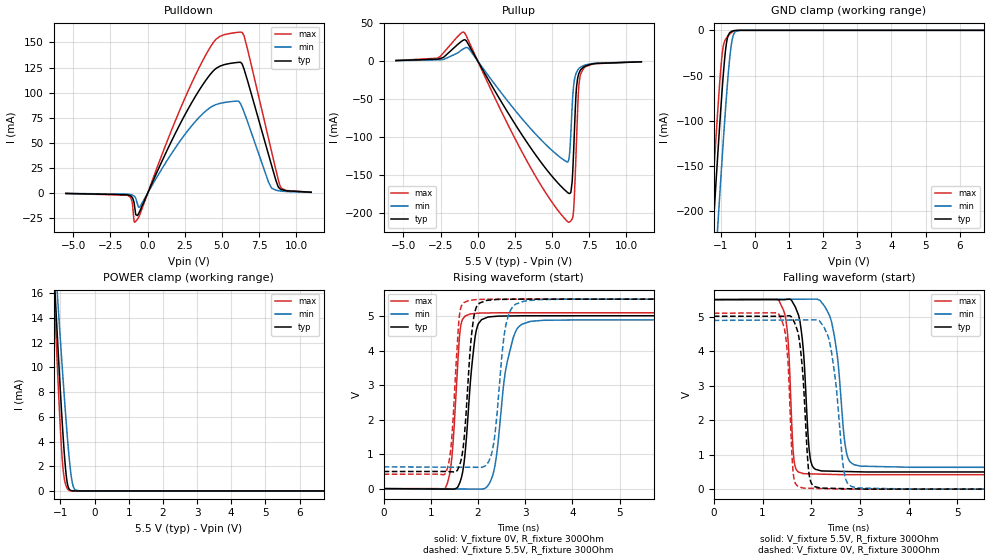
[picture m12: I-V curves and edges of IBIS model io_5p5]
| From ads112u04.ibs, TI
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|   io_5p5 Model
[Model]   io_5p5
Model_type   I/O
Polarity   Non-Inverting
Enable   Active-Low
Vinl = 1.65
Vinh = 3.85
Vmeas = 2.75
Vref = 0
Cref = 2pF
Rref = 100000
|   typ   min   max
C_comp   1.31716E-12   1.299E-12   1.3233E-12
|C_comp_pullup   9.8999E-13   9.67468E-13   1.02241E-12
|C_comp_pulldown   9.99226E-13   9.80937E-13   1.00378E-12
[Model spec]
|subparameter
Vinl   1.65   1.6497   1.6503
Vinh   3.85   3.8493   3.8507
| Where Nom  PVT is Nominal Process, 5.5V, 27C
|   Fast PVT is Strong Process,  5.501V, -40C
|   Slow PVT is Weak Process,   5.499, 125C
[Voltage Range]   5.5   5.499   5.501
[Temperature Range]   27   125   -40
[Pullup Reference]   5.5   5.499   5.501
[Pulldown Reference]   -0   -0   -0
[Power Clamp Reference]   5.5   5.499   5.501
[GND Clamp Reference]   0   0   0
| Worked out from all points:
|   slope of the pulldown table from 0 to 0.825 V, typ, clamps not added: 30.1 ohm
|   slope of the pullup table from 0 to 0.825 V, typ, clamps not added: 29 ohm
|   GND clamp passes 1 mA (typ) near -0.67 V on its own axis
|   POWER clamp passes 1 mA (typ) near -0.82 V on its own axis
|   falling waveform, V_fixture 5.5V, R_fixture 300Ohm: 20-80 % time 134ps typ, 206ps min, 99.9ps max; typ from 5.5 V to 0.497 V
|   rising waveform, V_fixture 0V, R_fixture 300Ohm: 20-80 % time 180ps typ, 269ps min, 138ps max; typ from 0 V to 5.02 V
|   rising waveform, V_fixture 5.5V, R_fixture 300Ohm: 20-80 % time 158ps typ, 202ps min, 133ps max; typ from 0.497 V to 5.5 V
|   falling waveform, V_fixture 0V, R_fixture 300Ohm: 20-80 % time 137ps typ, 209ps min, 102ps max; typ from 5.02 V to 0 V
[Pulldown]
|   Voltage   I(typ)   I(min)   I(max)
-5.5V     -139.3uA   -99uA      -151.9uA
-1.375V   -1.389mA   -810uA     -1.838mA
-995.5mV  -5.059mA   -1.917mA   -13.97mA
-797.5mV  -21.25mA   -4.806mA   -27.92mA
-517mV    -17.41mA   -13.24mA   -20.88mA
3.938V    112.8mA    82.15mA    138.3mA
4.862V    126.3mA    89.35mA    155.9mA
6.248V    130.2mA    89.06mA    160.2mA
6.495V    122.9mA    80.2mA     155.9mA
8.129V    38.5mA     11.1mA     54.47mA
8.921V    4.291mA    2.335mA    6.881mA
11V       1.086mA    904uA      1.089mA
[GND Clamp]
|   Voltage   I(typ)   I(min)   I(max)
-5.5V     -3.028A    -3.1A      -2.983A
-1.359V   -306.6mA   -386.8mA   -256.2mA
-1.243V   -234.4mA   -314.6mA   -184mA
-1.21V    -214.1mA   -294.2mA   -163.7mA
-1.078V   -134.5mA   -213.7mA   -85.68mA
-946mV    -61.21mA   -136.3mA   -23.61mA
-880mV    -30.87mA   -99.68mA   -11.73mA
-814mV    -10.85mA   -65.7mA    -7.744mA
-731.5mV  -2.627mA   -29.97mA   -4.178mA
-649mV    -712.3uA   -8.24mA    -1.554mA
-385mV    -967.4nA   -10.5uA    -935.9nA
11V       0A         0A         0A
[Pullup]
|   Voltage   I(typ)   I(min)   I(max)
-5.5V     607.8uA    492.8uA    650.8uA
-2.712V   2.442mA    1.477mA    3.672mA
-913mV    27.96mA    16.59mA    37.83mA
3.311V    -107.4mA   -83.78mA   -132.1mA
6.133V    -174.7mA   -129mA     -212.7mA
6.347V    -159.6mA   -60.35mA   -208.5mA
6.446V    -119.5mA   -32.8mA    -196.7mA
6.644V    -34.18mA   -14.75mA   -103.8mA
6.776V    -17.96mA   -10.57mA   -38.77mA
6.925V    -11.55mA   -7.969mA   -16.76mA
7.816V    -3.605mA   -3.152mA   -3.82mA
11V       -1.024mA   -975.5uA   -1.008mA
[POWER Clamp]
|   Voltage   I(typ)   I(min)   I(max)
-5.5V     270.1mA    226.1mA    321.7mA
-1.21V    19.05mA    21.23mA    17.88mA
-1.144V   15.48mA    18.34mA    13.59mA
-1.078V   12mA       15.51mA    9.461mA
-995.5mV  7.871mA    12.06mA    4.795mA
-929.5mV  4.843mA    9.381mA    2.021mA
-830.5mV  1.306mA    5.6mA      391.6uA
-731.5mV  107.1uA    2.383mA    34.68uA
-682mV    25.65uA    1.201mA    8.004uA
-616mV    3.994uA    316uA      953.9nA
-451mV    5.207nA    3.692uA    0A
11V       0A         0A         0A
[Ramp]
R_load = 300
|   typ   min   max
dV/dt_r   3.01089/1.80154e-10   2.93831/2.68594e-10   3.06275/1.37179e-10
dV/dt_f   3.00189/1.33627e-10   2.92036/2.05873e-10   3.04962/9.9851e-11
[Falling Waveform]
V_fixture = 5.5V
V_fixture_min = 5.499V
V_fixture_max = 5.501V
R_fixture = 300Ohm
C_fixture = 0F
|   Time   V(typ)   V(min)   V(max)
0s        5.5V       5.499V     5.501V
1.339ns   5.499V     5.509V     5.467V
1.51ns    5.509V     5.51V      4.564V
1.652ns   5.339V     5.511V     782.7mV
1.846ns   3.884V     5.512V     449.1mV
2.021ns   678.2mV    5.514V     442.6mV
2.415ns   522.3mV    4.864V     428mV
2.725ns   512.1mV    1.044V     419.7mV
3.014ns   502.7mV    667.1mV    419.7mV
50ns      496.9mV    631.7mV    418.3mV
[Rising Waveform]
V_fixture = 0V
V_fixture_min = 0V
V_fixture_max = 0V
R_fixture = 300Ohm
C_fixture = 0F
|   Time   V(typ)   V(min)   V(max)
0s        -331.9nV   -94.64nV   -82.16nV
1.307ns   -12.66mV   -8.387mV   15.08mV
1.444ns   -13.99mV   -9.268mV   890.3mV
1.571ns   46.68mV    -10.08mV   3.642V
1.671ns   462.9mV    -10.72mV   4.911V
2.03ns    4.827V     -13.03mV   5.094V
2.329ns   4.995V     480.3mV    5.1V
2.758ns   5.013V     4.431V     5.104V
3.389ns   5.017V     4.885V     5.104V
50ns      5.018V     4.897V     5.105V
[Rising Waveform]
V_fixture = 5.5V
V_fixture_min = 5.499V
V_fixture_max = 5.501V
R_fixture = 300Ohm
C_fixture = 0F
|   Time   V(typ)   V(min)   V(max)
0s        496.9mV    631.7mV    418.3mV
1.307ns   497.8mV    623.1mV    436mV
1.428ns   490.2mV    622.3mV    1.23V
1.562ns   534.1mV    621.4mV    4.228V
1.647ns   873.9mV    620.9mV    5.302V
1.999ns   5.332V     618.5mV    5.491V
2.296ns   5.476V     1.066V     5.497V
2.636ns   5.494V     4.991V     5.5V
3.267ns   5.499V     5.485V     5.5V
50ns      5.5V       5.499V     5.501V
[Falling Waveform]
|Gnd
V_fixture = 0V
V_fixture_min = 0V
V_fixture_max = 0V
R_fixture = 300Ohm
C_fixture = 0F
|   Time   V(typ)   V(min)   V(max)
0s        5.018V     4.897V     5.105V
1.339ns   5.017V     4.906V     5.069V
1.498ns   5.026V     4.908V     4.139V
1.636ns   4.89V      4.909V     405.6mV
1.84ns    3.084V     4.91V      30.31mV
2.008ns   158.4mV    4.911V     24.11mV
2.369ns   25.85mV    4.322V     10.79mV
2.672ns   16.09mV    520.1mV    1.474mV
2.971ns   6.421mV    34.16mV    1.473mV
50ns      -25.35nV   -91.71nV   -155.6nV
